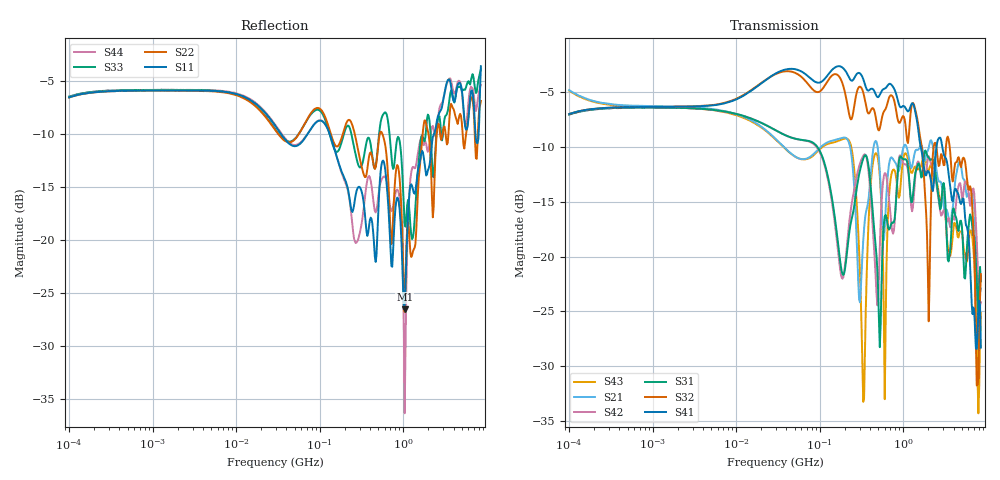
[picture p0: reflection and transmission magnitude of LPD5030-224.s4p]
# MHz S MA R 50
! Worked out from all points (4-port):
!   498 points, 100 kHz to 8.5 GHz, reference 50 ohm
!   strongest paths, dB at 100 kHz, 1.698 MHz, 29.49 MHz, 500.7 MHz, 8.5 GHz:
!     S41: -7.0, -6.3, -3.3, -5.4, -28.3
!     S32: -7.0, -6.3, -3.3, -8.4, -21.6
!     S31: -7.0, -6.4, -8.4, -23.1, -22.2
!     S42: -7.0, -6.4, -8.4, -24.0, -24.2
!     S21: -4.8, -6.3, -9.2, -10.3, -22.9
!     S43: -4.8, -6.4, -9.3, -11.1, -25.1
!   lowest |S11| = -26.6 dB at 1.04 GHz (marker M1), VSWR 1.10, Z = 53.5 + j3.42 ohm
!   |S11| at or under -10 dB: 34.58 MHz to 71.37 MHz (36.8 MHz wide, 69.5 % of centre); 132.1 MHz to 2.329 GHz (2.197 GHz wide, 179 % of centre); 7.336 GHz to 7.983 GHz (647.4 MHz wide, 8.45 % of centre)
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0.1  0.4722 20.1  0.5767 -16.9  0.4459 -158.7  0.448 21.7
     0.5767 -16.9  0.4709 20.1  0.4479 21.8  0.4462 -159.0
     0.4459 -158.7  0.4479 21.8  0.4759 20.1  0.5729 -17.0
     0.448 21.7  0.4462 -159.0  0.5729 -17.0  0.4753 20.2
215.0626  0.1779 -66.6  0.3427 7.8  0.1099 114.2  0.6798 -41.9
          0.3427 7.8  0.3654 -39.7  0.4909 -53.0  0.1198 110.6
          0.1099 114.2  0.4909 -53.0  0.3471 -36.5  0.3448 5.0
          0.6798 -41.9  0.1198 110.6  0.3448 5.0  0.1742 -68.7
331.9048  0.1553 -74.7  0.1181 25.2  0.2803 -0.9  0.6472 -64.1
          0.1181 25.2  0.2076 -66.2  0.5621 -65.3  0.289 -5.4
          0.2803 -0.9  0.5621 -65.3  0.2387 -39.8  0.02177 -29.0
          0.6472 -64.1  0.289 -5.4  0.02177 -29.0  0.1354 -28.5
1039.755  0.04702 42.8  0.3244 -114.9  0.2786 -116.9  0.4841 -168.3
          0.3244 -114.9  0.04582 -146.4  0.4234 -164.4  0.264 -123.3
          0.2786 -116.9  0.4234 -164.4  0.1198 -175.3  0.2947 -106.9
          0.4841 -168.3  0.264 -123.3  0.2947 -106.9  0.01519 -130.7
3111.8  0.4918 -9.2  0.1627 -59.9  0.2064 -81.7  0.2877 -85.7
        0.1627 -59.9  0.3442 -24.5  0.2622 -46.9  0.1602 -61.5
        0.2064 -81.7  0.2622 -46.9  0.3721 -15.5  0.1797 -71.9
        0.2877 -85.7  0.1602 -61.5  0.1797 -71.9  0.4883 -13.8
4588.001  0.5489 179.1  0.2665 129.2  0.131 107.8  0.1918 79.7
          0.2665 129.2  0.3707 -171.8  0.2848 106.7  0.2101 124.7
          0.131 107.8  0.2848 106.7  0.5275 174.0  0.1224 126.8
          0.1918 79.7  0.2101 124.7  0.1224 126.8  0.5655 171.3
8500  0.6625 -9.4  0.07163 -70.0  0.0773 -18.6  0.03849 10.2
      0.07163 -70.0  0.4538 -28.5  0.08324 62.4  0.06191 -32.3
      0.0773 -18.6  0.08324 62.4  0.6398 -44.0  0.05538 46.3
      0.03849 10.2  0.06191 -32.3  0.05538 46.3  0.5404 -36.0
